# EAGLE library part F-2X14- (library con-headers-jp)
FEMALE HEADER
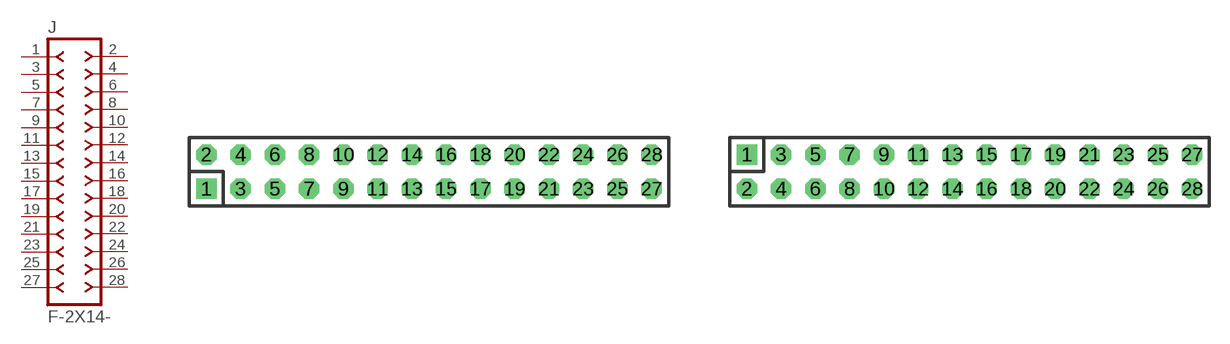
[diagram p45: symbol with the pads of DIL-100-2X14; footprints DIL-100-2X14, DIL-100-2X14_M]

Designator prefix J

## F-2X14-DIL-100  [DIL-100-2X14]
1  1  pas
2  2  pas
3  3  pas
4  4  pas
5  5  pas
6  6  pas
7  7  pas
8  8  pas
9  9  pas
10  10  pas
11  11  pas
12  12  pas
13  13  pas
14  14  pas
15  15  pas
16  16  pas
17  17  pas
18  18  pas
19  19  pas
20  20  pas
21  21  pas
22  22  pas
23  23  pas
24  24  pas
25  25  pas
26  26  pas
27  27  pas
28  28  pas

## F-2X14-DIL-100_M  [DIL-100-2X14_M]
Pads as for DIL-100-2X14

## F-2X14-DIL-2MM  [DIL-2MM-2X14]
Pads as for DIL-100-2X14

## F-2X14-DIL-2MM_M  [DIL-2MM-2X14_M]
Pads as for DIL-100-2X14

## F-2X14-71991  [71991-28]
Pads as for DIL-100-2X14

## Footprint DIL-100-2X14 (pad centres in mm)
PIN HEADER - 0.1"
drill 1.016 square: 1 -16.51,-1.27
drill 1.016 octagon: 2 -16.51,1.27; 3 -13.97,-1.27; 4 -13.97,1.27; 5 -11.43,-1.27; 6 -11.43,1.27; 7 -8.89,-1.27; 8 -8.89,1.27; 9 -6.35,-1.27; 10 -6.35,1.27; 11 -3.81,-1.27; 12 -3.81,1.27; 13 -1.27,-1.27; 14 -1.27,1.27; 15 1.27,-1.27; 16 1.27,1.27; 17 3.81,-1.27; 18 3.81,1.27; 19 6.35,-1.27; 20 6.35,1.27; 21 8.89,-1.27; 22 8.89,1.27; 23 11.43,-1.27; 24 11.43,1.27; 25 13.97,-1.27; 26 13.97,1.27; 27 16.51,-1.27; 28 16.51,1.27

## Footprint DIL-100-2X14_M (pad centres in mm)
PIN HEADER - MIRRORED 0.1"
drill 1.016 square: 1 -16.51,1.27
drill 1.016 octagon: 2 -16.51,-1.27; 3 -13.97,1.27; 4 -13.97,-1.27; 5 -11.43,1.27; 6 -11.43,-1.27; 7 -8.89,1.27; 8 -8.89,-1.27; 9 -6.35,1.27; 10 -6.35,-1.27; 11 -3.81,1.27; 12 -3.81,-1.27; 13 -1.27,1.27; 14 -1.27,-1.27; 15 1.27,1.27; 16 1.27,-1.27; 17 3.81,1.27; 18 3.81,-1.27; 19 6.35,1.27; 20 6.35,-1.27; 21 8.89,1.27; 22 8.89,-1.27; 23 11.43,1.27; 24 11.43,-1.27; 25 13.97,1.27; 26 13.97,-1.27; 27 16.51,1.27; 28 16.51,-1.27

## Footprint DIL-2MM-2X14 (pad centres in mm)
PIN HEADER - 2MM
drill 0.711 square: 1 -13,-1
drill 0.711: 2 -13,1; 3 -11,-1; 4 -11,1; 5 -9,-1; 6 -9,1; 7 -7,-1; 8 -7,1; 9 -5,-1; 10 -5,1; 11 -3,-1; 12 -3,1; 13 -1,-1; 14 -1,1; 15 1,-1; 16 1,1; 17 3,-1; 18 3,1; 19 5,-1; 20 5,1; 21 7,-1; 22 7,1; 23 9,-1; 24 9,1; 25 11,-1; 26 11,1; 27 13,-1; 28 13,1

## Footprint DIL-2MM-2X14_M (pad centres in mm)
PIN HEADER - MIRRORED 2MM
drill 0.711 square: 1 -13,1
drill 0.711: 2 -13,-1; 3 -11,1; 4 -11,-1; 5 -9,1; 6 -9,-1; 7 -7,1; 8 -7,-1; 9 -5,1; 10 -5,-1; 11 -3,1; 12 -3,-1; 13 -1,1; 14 -1,-1; 15 1,1; 16 1,-1; 17 3,1; 18 3,-1; 19 5,1; 20 5,-1; 21 7,1; 22 7,-1; 23 9,1; 24 9,-1; 25 11,1; 26 11,-1; 27 13,1; 28 13,-1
